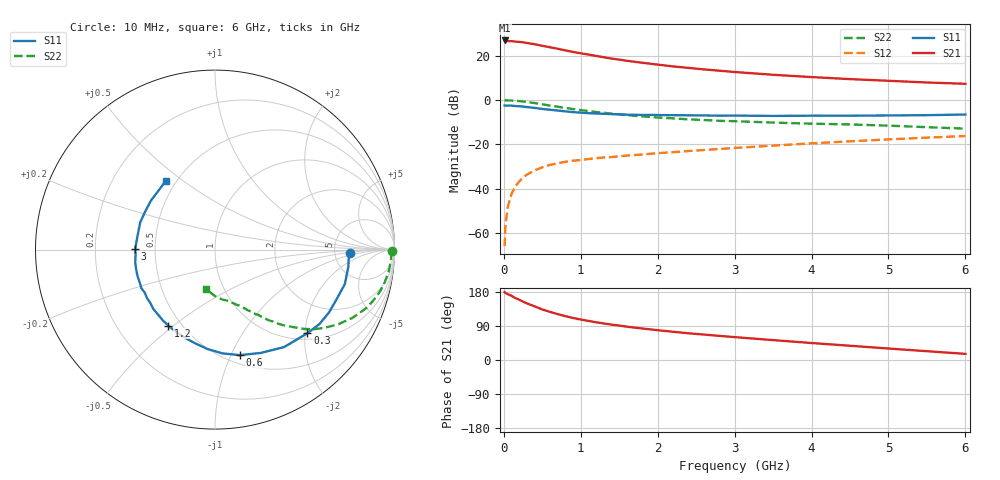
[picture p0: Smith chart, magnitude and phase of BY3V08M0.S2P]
! SIEMENS Small Signal Semiconductors
! BFY420
! Si NPN RF SIEGET Grounded Emitter Transistor in MICRO-X
! VCE = 3 V  IC = 8 mA
! Common Emitter S-Parameters:  October  1996
# GHz  S  MA  R  50
!  f  S11  S21  S12  S22
! GHz  MAG  ANG  MAG  ANG  MAG  ANG  MAG  ANG
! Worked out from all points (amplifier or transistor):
!   36 points, 10 MHz to 6 GHz, reference 50 ohm
!   highest |S21| = 26.9 dB at 10 MHz (marker M1)
!   |S21| within 3 dB of that: start of sweep to 590.3 MHz
!   unconditionally stable (mu >= 1): 2.712 GHz to end of sweep
!   at 250 MHz: K = 0.16, MSG = 30.5 dB, |S12| = -35.0 dB
!   at 1.4 GHz: K = 0.68, MSG = 22.2 dB, |S12| = -25.7 dB
!   at 6 GHz: K = 1.11, MAG = 9.8 dB, |S12| = -16.2 dB
!   S11 on the Smith chart (normalised r, x): 10 MHz: 6.97, -0.67; 300 MHz: 1.15, -2.06; 600 MHz: 0.58, -1.08; 1.2 GHz: 0.43, -0.48; 3 GHz: 0.38, +0.00; 6 GHz: 0.44, +0.43
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0.01  0.7512 -1.6  22.22 179.2  0.0005 74.9  0.9848 -0.6
0.02  0.7468 -3.0  21.94 177.0  0.0014 80.4  0.9814 -1.4
0.05  0.7488 -7.4  21.52 173.8  0.0038 85.8  0.9829 -3.5
0.1  0.7484 -14.9  21.42 169.5  0.0076 79.3  0.975 -7.4
0.15  0.7327 -21.7  20.92 163.3  0.0112 76.6  0.9625 -11.0
0.2  0.7253 -28.9  20.63 159.2  0.0145 74.6  0.9482 -14.3
0.25  0.7143 -35.6  20.18 154.0  0.0178 72.4  0.9265 -17.8
0.3  0.6944 -42.1  19.51 149.4  0.0207 69.6  0.9061 -20.9
0.4  0.6659 -54.6  18.27 141.6  0.0258 64.4  0.8551 -26.4
0.5  0.6297 -66.1  16.82 133.3  0.0302 60.8  0.8028 -31.2
0.6  0.6042 -76.7  15.62 127.0  0.0343 57.2  0.7526 -35.3
0.8  0.5558 -94.2  13.25 115.7  0.0403 51.8  0.6645 -41.7
0.9  0.5342 -101.8  12.24 110.9  0.0427 50.7  0.6265 -43.9
1.1  0.5057 -116.2  10.67 103.1  0.0466 48.5  0.5641 -48.2
1.2  0.4968 -121.6  9.942 99.5  0.0487 47.9  0.5373 -49.9
1.6  0.4666 -141.0  7.714 87.9  0.0558 45.8  0.4563 -55.2
2.2  0.4563 -161.1  5.759 74.5  0.0666 44.9  0.3861 -61.4
3  0.4454 179.8  4.307 60.4  0.0828 43.3  0.333 -68.1
3.5  0.4383 169.2  3.724 52.5  0.0935 41.4  0.3101 -72.3
4.5  0.4431 151.3  2.973 37.6  0.1169 36.4  0.2813 -81.5
5.5  0.4558 133.2  2.494 23.2  0.1416 29.3  0.244 -94.7
6  0.4712 125.5  2.333 16.2  0.154 25.4  0.2264 -103.0
